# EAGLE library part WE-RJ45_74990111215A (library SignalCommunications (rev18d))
Order Code 74990111215A Design THT xBase-T 10/100 Base-T Ports 1x1 Application Standard HPLE Tab Position Down LED (Left-Right) YELLOW-GREEN EMI Fingers YES Details see: http://katalog.we-online.de/en/pbs/WE-LAN_RJ45/74990111215A? Updated by Yingchun Shan 2016-08-29 2016(C) Würth Elektronik
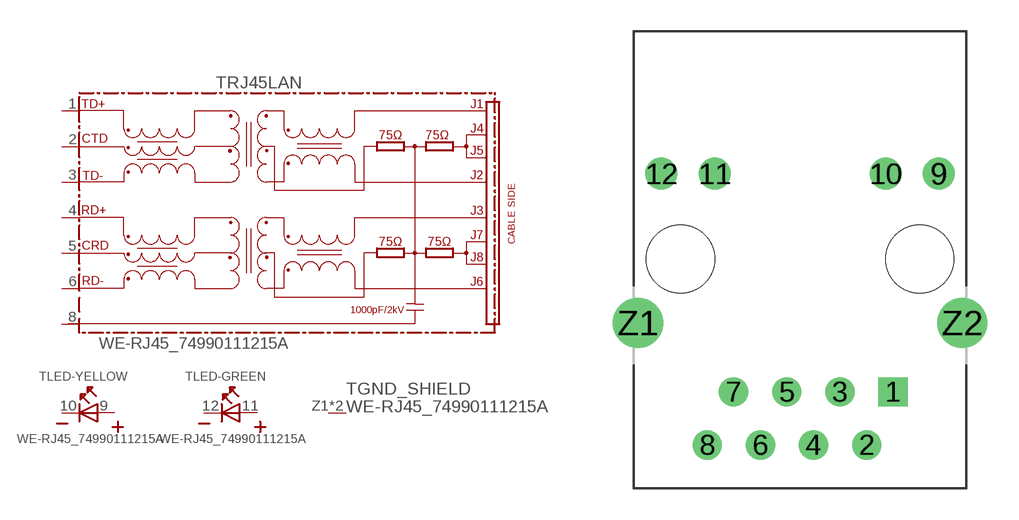
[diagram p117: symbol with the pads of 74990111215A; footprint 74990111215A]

Designator prefix T; gates RJ45LAN=74990111215A LED-YELLOW=LED-2PIN LED-GREEN=LED-2PIN GND_SHIELD=GND_PIN

## WE-RJ45_74990111215A (COMPANY-URL: http://www.we-online.de; CREATED-BY: Christin Zierenner; CREATED-DATE: AUG 2012; DATASHEET-URL: http://katalog.we-online.de/kataloge/eisos/media/pdf/74990111215A.pdf; MANUFACTURER: Würth Elektronik eiSos GmbH)  [74990111215A]
1  RJ45LAN:TD+
2  RJ45LAN:CTD
3  RJ45LAN:TD-
4  RJ45LAN:RD+
5  RJ45LAN:CRD
6  RJ45LAN:RD-
8  RJ45LAN:SH  pwr
9  LED-YELLOW:A  pas
10  LED-YELLOW:K  pas
11  LED-GREEN:A  pas
12  LED-GREEN:K  pas
Z1  GND_SHIELD:1  pwr
Z2  GND_SHIELD:1  pwr

## Footprint 74990111215A (pad centres in mm)
MAX HEIGHT=13.74mm PORTS----1X1 LED --YES
drill 0.89 square: 1 4.44,-6.35
drill 0.89: 2 3.18,-8.89; 3 1.9,-6.35; 4 0.64,-8.89; 5 -0.64,-6.35; 6 -1.9,-8.89; 7 -3.18,-6.35; 8 -4.44,-8.89
drill 1.02: 9 6.625,4.08; 10 4.085,4.08; 11 -4.085,4.08; 12 -6.625,4.08
drill 1.6: Z1 -7.745,-3.05; Z2 7.745,-3.05
hole 3.25 at 5.715,0
hole 3.25 at -5.715,0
